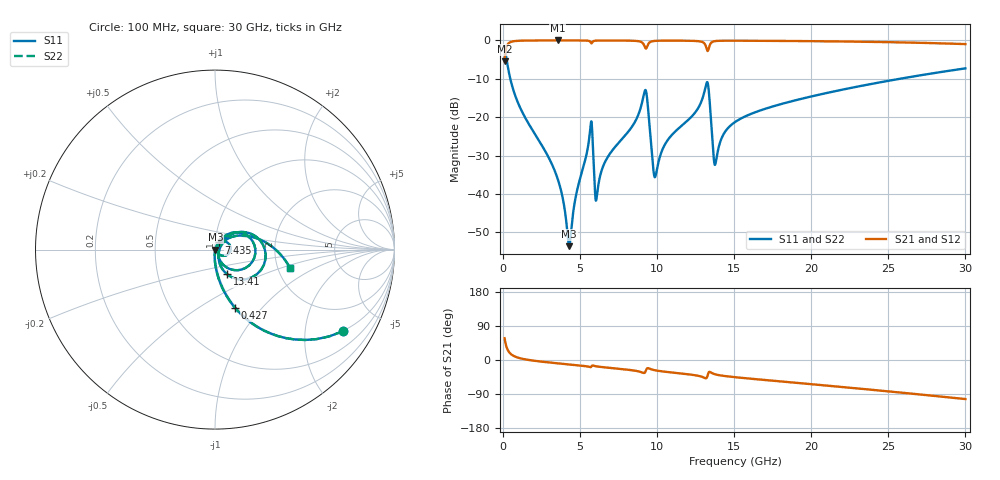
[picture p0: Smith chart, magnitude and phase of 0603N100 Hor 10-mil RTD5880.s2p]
# GHz S MA R 50
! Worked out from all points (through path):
!   3201 points, 100 MHz to 30 GHz, reference 50 ohm
!   highest |S21| = -0.02 dB at 3.548 GHz (marker M1); lowest = -5.4 dB at 100 MHz (marker M2)
!   group delay of S21, straight-line fit = 9.98 ps
!   lowest |S11| = -53.6 dB at 4.286 GHz (marker M3), VSWR 1.00, Z = 50.2 - j0.0559 ohm
!   |S11| at or under -10 dB: 468.9 MHz to 25.74 GHz (25.28 GHz wide, 193 % of centre)
!   |S22| runs from -53.6 to -1.5 dB; largest |S21 - S12| = 0
!   S11 on the Smith chart (normalised r, x): 100 MHz: 0.99, -3.14; 427 MHz: 0.99, -0.73; 7.435 GHz: 1.04, +0.08; 13.41 GHz: 1.10, -0.31; 30 GHz: 2.34, -0.60
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0.1  0.8449 -32.6  0.5347 57.4  0.5347 57.4  0.8449 -32.6
0.4270312  0.3443 -70.9  0.9383 19.0  0.9383 19.0  0.3443 -70.9
1.286656  0.1122 -86.5  0.9926 2.9  0.9926 2.9  0.1122 -86.5
3.547844  0.01565 -92.2  0.998 -8.8  0.998 -8.8  0.01565 -92.2
4.286  0.002087 -15.5  0.9979 -11.7  0.9979 -11.7  0.002087 -15.5
5.089563  0.01854 65.6  0.9967 -14.9  0.9967 -14.9  0.01854 65.6
5.668875  0.0747 35.3  0.9544 -18.9  0.9544 -18.9  0.0747 35.3
6.08  0.00914 29.9  0.9936 -17.0  0.9936 -17.0  0.00914 29.9
6.565875  0.02484 62.8  0.9962 -19.3  0.9962 -19.3  0.02484 62.8
7.434844  0.04479 62.6  0.9953 -22.8  0.9953 -22.8  0.04479 62.6
9.2195  0.2247 0.8  0.8037 -32.0  0.8037 -32.0  0.2247 0.8
9.378344  0.151 -48.5  0.863 -21.5  0.863 -21.5  0.151 -48.5
9.780125  0.01861 -31.4  0.9813 -26.4  0.9813 -26.4  0.01861 -31.4
10.06978  0.0252 37.8  0.9895 -28.6  0.9895 -28.6  0.0252 37.8
13.18125  0.2692 5.5  0.8159 -48.0  0.8159 -48.0  0.2692 5.5
13.41484  0.1518 -64.0  0.8686 -31.4  0.8686 -31.4  0.1518 -64.0
13.63909  0.03508 -56.1  0.9668 -36.0  0.9668 -36.0  0.03508 -56.1
13.77925  0.02459 -1.6  0.9799 -37.9  0.9799 -37.9  0.02459 -1.6
15.05  0.08635 41.1  0.9907 -45.3  0.9907 -45.3  0.08635 41.1
20.03956  0.1869 24.6  0.9773 -63.9  0.9773 -63.9  0.1869 24.6
25.01978  0.298 6.1  0.9486 -82.9  0.9486 -82.9  0.298 6.1
30  0.4322 -13.9  0.8948 -103.1  0.8948 -103.1  0.4322 -13.9
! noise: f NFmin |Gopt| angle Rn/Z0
0.1  0.0003221  0.926  0.5424  0.0009648
3.417  0.003619  0.7903  9.364  0.003534
6.743  0.006952  0.786  18.31  0.006512
10.06  0.01495  0.8474  27.25  0.0197
13.39  0.07335  0.9565  36.07  0.3438
16.7  0.01291  0.7303  44.33  0.008213
20.03  0.0145  0.7175  52.54  0.008216
23.35  0.01655  0.7153  60.54  0.008639
26.67  0.01881  0.7172  68.36  0.009113
30  0.0213  0.722  75.96  0.00959
